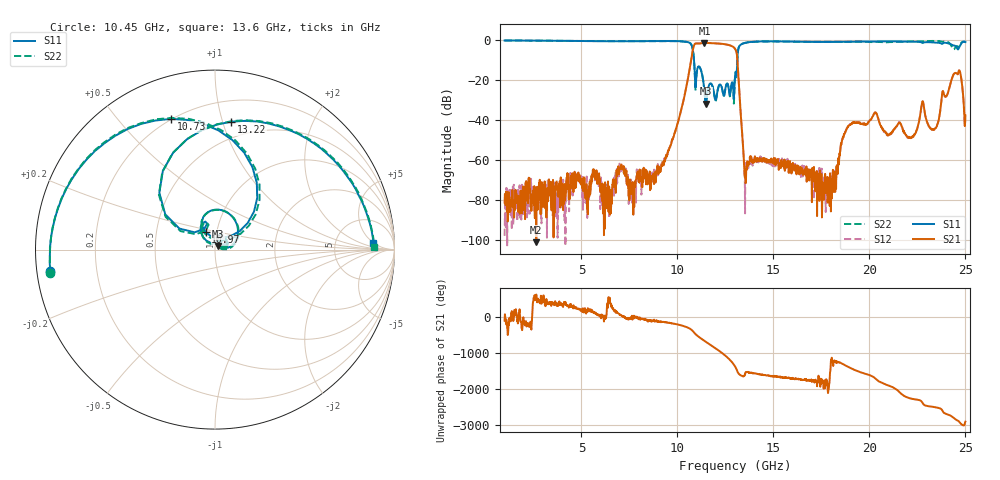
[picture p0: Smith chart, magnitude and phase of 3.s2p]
!The following data was pulled from an Agilent PNA
!This sNp file was generated from the data in the RF Test software
!NOTE:  Smoothing/Math/Corrections applied on any given trace ARE included in the data saved here
# MHz S dB R 50
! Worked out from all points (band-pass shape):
!   1601 points, 1 GHz to 25 GHz, reference 50 ohm
!   highest |S21| = -1.22 dB at 11.41 GHz (marker M1); lowest = -101.1 dB at 2.65 GHz (marker M2)
!   |S21| within 3 dB of the highest: 10.82 GHz to 13 GHz (2.188 GHz wide, 18.4 % of centre)
!   lowest |S11| = -31.6 dB at 11.48 GHz (marker M3), VSWR 1.05, Z = 51.6 + j2.15 ohm
!   |S11| at or under -10 dB: 10.87 GHz to 13.12 GHz (2.25 GHz wide, 18.8 % of centre)
!   |S22| runs from -32.3 to 0.0 dB; largest |S21 - S12| = 0.006
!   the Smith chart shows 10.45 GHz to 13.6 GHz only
!   S11 on the Smith chart (normalised r, x): 10.45 GHz: 0.04, -0.07; 10.73 GHz: 0.20, +0.70; 10.97 GHz: 0.89, +0.17; 13.22 GHz: 0.36, +1.07; 13.6 GHz: 14, +5
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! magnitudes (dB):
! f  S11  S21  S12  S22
! 1 GHz  0.0  -81.2  -97.7  0.0
! 2.65 GHz  -0.1  -101.1  -80.9  -0.1
! 5.005 GHz  -0.3  -69.8  -70.0  -0.3
! 6.43 GHz  -0.4  -80.1  -83.5  -0.3
! 9.01 GHz  -0.3  -66.9  -64.5  -0.3
! 10.45 GHz  -0.7  -24.1  -24.1  -0.7
! 10.73 GHz  -2.3  -8.5  -8.4  -2.3
! 10.97 GHz  -19.2  -1.5  -1.5  -19.7
! 11.41 GHz  -25.6  -1.2  -1.2  -25.6
! 11.48 GHz  -31.6  -1.2  -1.2  -32.3
! 13 GHz  -17.9  -4.2  -4.2  -18.4
! 13.22 GHz  -2.9  -26.0  -25.9  -2.8
! 13.6 GHz  -1.1  -64.5  -61.7  -1.0
! 17 GHz  -0.7  -80.9  -64.1  -0.7
! 17.93 GHz  -0.7  -82.8  -76.5  -0.6
! 19.09 GHz  -0.6  -41.5  -41.3  -0.6
! 21.01 GHz  -0.4  -47.1  -47.3  -0.9
! 22.24 GHz  -0.6  -47.9  -48.5  -0.4
! 22.77 GHz  -1.2  -30.5  -30.6  -0.5
! 23.39 GHz  -1.0  -44.4  -44.3  -0.3
! 24.59 GHz  -4.4  -17.0  -17.0  -2.9
! 25 GHz  -0.8  -37.5  -37.6  -0.6
